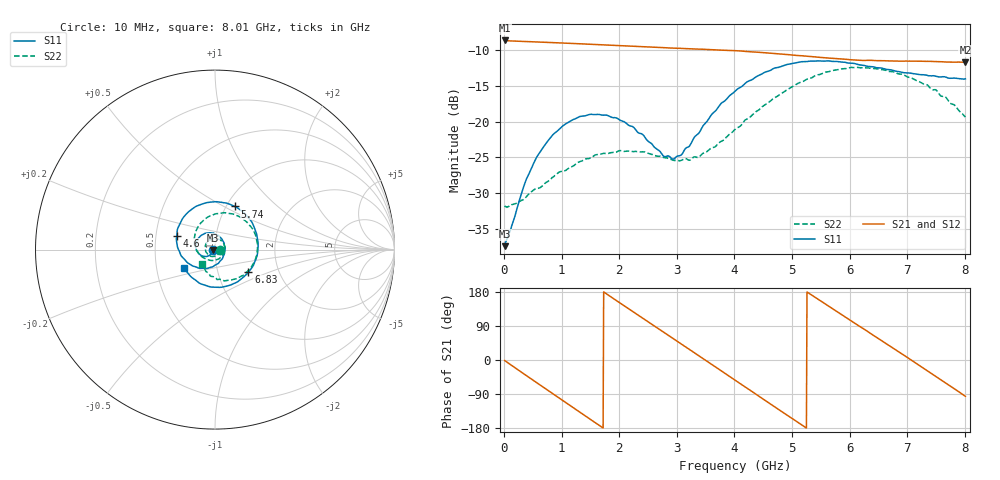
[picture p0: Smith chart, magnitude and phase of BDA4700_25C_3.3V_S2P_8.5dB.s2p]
!Agilent Technologies,E5071B,MY42404982,A.09.10
!Date: Mon Oct 20 18:06:34 2025
!Data & Calibration Information:
!Freq	S11:SOLT2(ON)	S21:SOLT2(ON)	S12:SOLT2(ON)	S22:SOLT2(ON)
# Hz S RI R 50
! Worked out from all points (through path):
!   801 points, 10 MHz to 8.01 GHz, reference 50 ohm
!   highest |S21| = -8.62 dB at 10 MHz (marker M1); lowest = -11.7 dB at 8.01 GHz (marker M2)
!   group delay of S21, straight-line fit = 282 ps
!   lowest |S11| = -37.5 dB at 10 MHz (marker M3), VSWR 1.03, Z = 48.7 - j0.158 ohm
!   |S11| at or under -10 dB: start of sweep to end of sweep
!   |S22| runs from -32.0 to -12.4 dB; largest |S21 - S12| = 0.0043
!   S11 on the Smith chart (normalised r, x): 10 MHz: 0.97, -0.00; 4.6 GHz: 0.64, +0.11; 5.74 GHz: 1.09, +0.57; 6.83 GHz: 1.40, -0.37; 8.01 GHz: 0.69, -0.15
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1e7  -0.0133 -0.00163  0.3707 -0.00808  0.3707 -0.00843  0.0257 -0.0013
3.6e8  -0.0248 -0.0272  0.2864 -0.2256  0.2862 -0.2258  0.0207 -0.0204
5.8e8  -0.0434 -0.0377  0.1743 -0.3172  0.1742 -0.3171  0.0109 -0.0322
9.5e8  -0.0834 -0.0276  -0.0603 -0.3517  -0.0603 -0.3517  -0.0233 -0.0375
1.35e9  -0.1077 0.0191  -0.2736 -0.2198  -0.2736 -0.22  -0.0527 -0.00532
1.64e9  -0.0945 0.0611  -0.3424 -0.0533  -0.3426 -0.0532  -0.0509 0.0294
1.93e9  -0.0577 0.0896  -0.3191 0.1225  -0.3192 0.1226  -0.0238 0.0559
2.32e9  0.00569 0.084  -0.1635 0.2935  -0.1635 0.2934  0.0254 0.0563
2.68e9  0.049 0.0399  0.0436 0.3284  0.0429 0.3282  0.0542 0.0181
2.96e9  0.0534 -0.0131  0.1921 0.265  0.192 0.2646  0.0504 -0.0182
3.37e9  0.00963 -0.0815  0.315 0.069  0.3153 0.069  0.0101 -0.0552
3.68e9  -0.0596 -0.1041  0.3007 -0.1049  0.3006 -0.1058  -0.0355 -0.0573
4.01e9  -0.1422 -0.0801  0.1889 -0.2513  0.1892 -0.2506  -0.0818 -0.0324
4.6e9  -0.2127 0.0779  -0.1208 -0.2775  -0.1203 -0.2778  -0.1127 0.0776
4.99e9  -0.1577 0.2007  -0.2617 -0.1326  -0.2621 -0.1335  -0.0655 0.1617
5.35e9  -0.0397 0.2624  -0.2815 0.0477  -0.2817 0.046  0.0279 0.2017
5.74e9  0.1099 0.2404  -0.1835 0.2074  -0.1834 0.2074  0.1457 0.1774
6.19e9  0.2241 0.1097  0.0126 0.2685  0.016 0.2693  0.2308 0.0598
6.68e9  0.2182 -0.077  0.2081 0.1662  0.2087 0.166  0.2073 -0.0878
6.83e9  0.1863 -0.1257  0.243 0.1073  0.2437 0.1056  0.1793 -0.1226
7.35e9  0.0182 -0.2104  0.2324 -0.1263  0.2325 -0.1265  0.0505 -0.1737
8.01e9  -0.1718 -0.1012  -0.0266 -0.2592  -0.0259 -0.2593  -0.0722 -0.08
